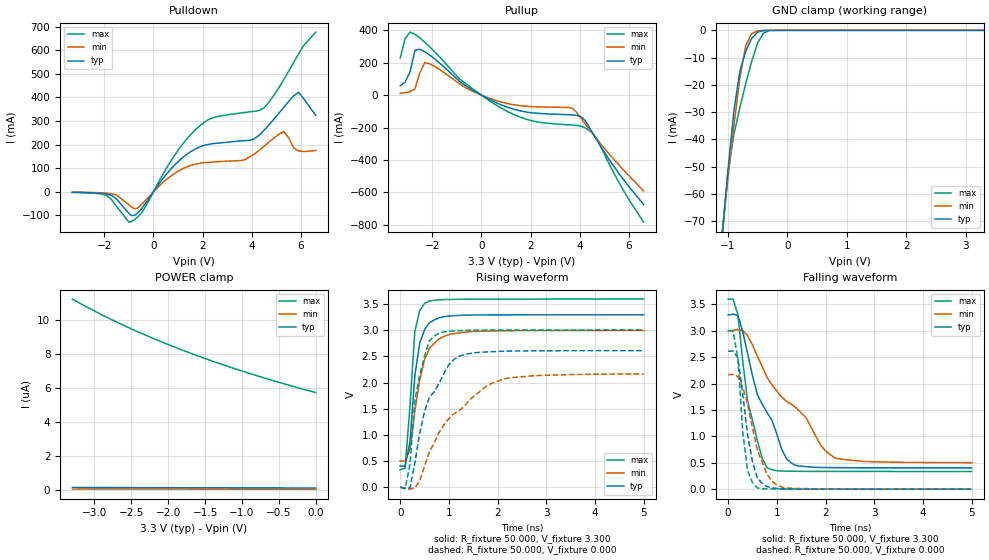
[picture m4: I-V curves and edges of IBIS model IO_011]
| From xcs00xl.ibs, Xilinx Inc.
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|   Model IO_011
[Model]   IO_011
Model_type   I/O
Polarity   Non-Inverting
Enable   Active-Low
Vinl =   0.800V
Vinh =   2.000V
Vmeas =   1.650V
Cref =  50.000pF
Rref =   1.000M
Vref =  0.000V
C_comp   5.300pF   3.500pF   6.800pF
[Temperature Range]   50.000   100.000   0.000
[Voltage Range]   3.300V   3.000V   3.600V
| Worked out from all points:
|   slope of the pulldown table from 0 to 0.495 V, typ, clamps not added: 7.07 ohm
|   slope of the pullup table from 0 to 0.495 V, typ, clamps not added: 12.6 ohm
|   GND clamp passes 1 mA (typ) near -0.52 V on its own axis
|   rising waveform, R_fixture 50.000, V_fixture 3.300: 20-80 % time 185ps typ, 288ps min, 145ps max; typ from 0.402 V to 3.3 V
|   rising waveform, R_fixture 50.000, V_fixture 0.000: 20-80 % time 542ps typ, 991ps min, 258ps max; typ from 0 V to 2.61 V
|   falling waveform, R_fixture 50.000, V_fixture 3.300: 20-80 % time 659ps typ, 1.19ns min, 341ps max; typ from 3.3 V to 0.403 V
|   falling waveform, R_fixture 50.000, V_fixture 0.000: 20-80 % time 242ps typ, 372ps min, 160ps max; typ from 2.61 V to 0.001 V
[Pulldown]
| voltage   I(typ)   I(min)   I(max)
-3.3V     -2.3mA     -1.8mA     -2.8mA
-1.9V     -9.7mA     -6.1mA     -16.3mA
-900mV    -100mA     -63.86mA   -127mA
-400mV    -59.92mA   -44.53mA   -76.62mA
700mV     94.99mA    66.07mA    129mA
1.6V      175mA      114mA      252mA
2.3V      202mA      125mA      309mA
3.6V      216mA      133mA      335mA
4.5V      261mA      193mA      356mA
5.3V      358mA      255mA      476mA
5.9V      422mA      173mA      584mA
6.6V      324mA      175mA      677mA
[Pullup]
| voltage   I(typ)   I(min)   I(max)
-3.3V     58.45mA    12.11mA    229mA
-3.1V     79.83mA    15.13mA    349mA
-2.9V     144mA      21.48mA    389mA
-2.7V     277mA      39.71mA    375mA
-2.5V     283mA      139mA      353mA
-2.1V     247mA      193mA      298mA
-800mV    74.73mA    60.76mA    89.48mA
900mV     -65.46mA   -46.11mA   -87.59mA
3.6V      -121mA     -77.38mA   -184mA
4V        -131mA     -132mA     -189mA
4.7V      -278mA     -272mA     -271mA
6.6V      -675mA     -591mA     -784mA
[GND_clamp]
| voltage   I(typ)   I(min)   I(max)
-3.3V     -539mA     -461mA     -635mA
-1.1V     -76.29mA   -74.81mA   -76.3mA
-1V       -51.66mA   -54.6mA    -52.25mA
-900mV    -29.77mA   -35.09mA   -38.23mA
-800mV    -15.1mA    -17.65mA   -28.49mA
-700mV    -7.645mA   -5.66mA    -19.53mA
-600mV    -2.968mA   -1.205mA   -11.34mA
-500mV    -649uA     -202uA     -4.68mA
-400mV    -83.34uA   -28.89uA   -976uA
-300mV    -8.303uA   -3.567uA   -95.2uA
3.3V      91.94nA    24.12nA    4.611uA
[POWER_clamp]
| voltage   I(typ)   I(min)   I(max)
-3.3V     126nA      27.82nA    11.23uA
-2.9V     121nA      27.69nA    10.3uA
-2.6V     117nA      27.29nA    9.671uA
-2.2V     113nA      27nA       8.903uA
-1.8V     109nA      25.98nA    8.207uA
-1.4V     104nA      25.34nA    7.571uA
-1V       101nA      24.85nA    6.988uA
-600mV    97.4nA     24.51nA    6.451uA
0V        91.93nA    23.77nA    5.718uA
[Ramp]
| variable   typ   min   max
dV/dt_r   1.567/0.517n   1.299/0.991n   1.805/0.280n
dV/dt_f   1.738/0.629n   1.497/1.169n   1.958/0.348n
R_load = 50.000
[Rising Waveform]
R_fixture = 50.000
V_fixture = 3.300
V_fixture_min = 3.000
V_fixture_max = 3.600
L_fixture = 0.000H
C_fixture = 0.000F
| time   V(typ)   V(min)   V(max)
0s        402mV      503mV      335mV
100ps     404mV      499mV      362mV
200ps     861mV      715mV      1.55V
300ps     2.127V     1.456V     2.977V
400ps     2.755V     2.052V     3.377V
500ps     3.013V     2.442V     3.515V
600ps     3.147V     2.656V     3.563V
800ps     3.239V     2.837V     3.584V
1.2ns     3.285V     2.95V      3.593V
5ns       3.298V     2.998V     3.598V
[Rising Waveform]
R_fixture = 50.000
V_fixture = 0.000
V_fixture_min = 0.000
V_fixture_max = 0.000
L_fixture = 0.000H
C_fixture = 0.000F
| time   V(typ)   V(min)   V(max)
0s        0V         0V         0V
100ps     -26.7mV    -19.53mV   -26.7mV
200ps     -16.57mV   -38.29mV   440mV
300ps     466mV      -13.62mV   1.653V
400ps     1.032V     124mV      2.145V
600ps     1.726V     675mV      2.8V
700ps     1.827V     849mV      2.892V
1.2ns     2.5V       1.459V     2.995V
2.1ns     2.599V     2.062V     3.006V
5ns       2.611V     2.165V     3.008V
[Falling Waveform]
R_fixture = 50.000
V_fixture = 3.300
V_fixture_min = 3.000
V_fixture_max = 3.600
L_fixture = 0.000H
C_fixture = 0.000F
| time   V(typ)   V(min)   V(max)
0s        3.3V       3V         3.6V
100ps     3.315V     3.008V     3.601V
200ps     3.291V     3.023V     3.307V
400ps     2.562V     2.907V     1.668V
600ps     1.79V      2.516V     918mV
800ps     1.448V     2.117V     404mV
1.1ns     755mV      1.745V     344mV
1.3ns     493mV      1.606V     340mV
2.2ns     406mV      590mV      337mV
5ns       403mV      504mV      336mV
[Falling Waveform]
R_fixture = 50.000
V_fixture = 0.000
V_fixture_min = 0.000
V_fixture_max = 0.000
L_fixture = 0.000H
C_fixture = 0.000F
| time   V(typ)   V(min)   V(max)
0s        2.613V     2.169V     3.009V
100ps     2.618V     2.173V     2.991V
200ps     2.486V     2.135V     2.482V
300ps     1.799V     1.931V     1.079V
400ps     1.032V     1.606V     350mV
500ps     522mV      1.157V     121mV
600ps     211mV      738mV      23.43mV
800ps     48.67mV    280mV      7.013mV
1.1ns     8.649mV    40.88mV    3.193mV
5ns       737uV      819uV      657uV
